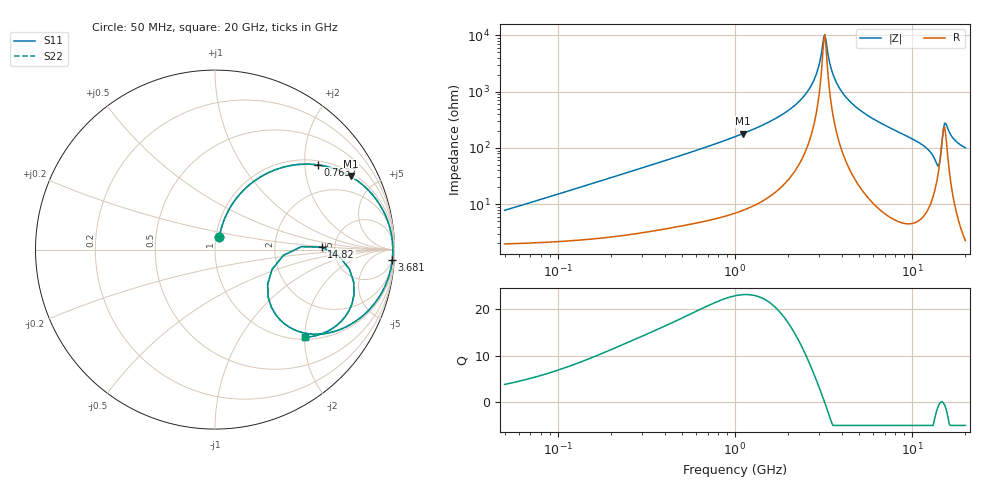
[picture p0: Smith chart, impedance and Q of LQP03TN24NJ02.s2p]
!Murata Part Number: LQP03TN24NJ02
!These Parameters are Measured in Series Mode Connection
!  o--[Z]--o
!Port1  Port2
!  o-------o
!Freq. Start=50[MHz] Stop=20[GHz], 401[Steps]
# Hz S RI R 50
!Freq.(Hz) S11(Real) S11(Imag) S21(Real) S21(Imag) S12(Real) S12(Imag) S22(Real) S22(Imag)
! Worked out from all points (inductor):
!   401 points, 50 MHz to 20 GHz, reference 50 ohm
!   read as one part in series: L = 23.9 nH near 51.52 MHz
!   highest Q = 23.2 at 1.111 GHz (marker M1), where L = 25.8 nH
!   self-resonance near 3.169 GHz
!   S11 on the Smith chart (normalised r, x): 50 MHz: 1.04, +0.15; 763.7 MHz: 1.11, +2.33; 3.681 GHz: 6, -32; 14.82 GHz: 3.94, +0.17; 20 GHz: 1.04, -2.01
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5e7  0.0246 0.072  0.9754 -0.072  0.9754 -0.072  0.0246 0.072
1.364002e8  0.0596 0.1864  0.9404 -0.1864  0.9404 -0.1864  0.0596 0.1864
3.721004e8  0.2461 0.4003  0.7539 -0.4003  0.7539 -0.4003  0.2461 0.4003
7.636728e8  0.572 0.472  0.428 -0.472  0.428 -0.472  0.572 0.472
1e9  0.7074 0.4337  0.2926 -0.4337  0.2926 -0.4337  0.7074 0.4337
1.110545e9  0.7557 0.4086  0.2443 -0.4086  0.2443 -0.4086  0.7557 0.4086
1.99176e9  0.9443 0.2021  0.0557 -0.2021  0.0557 -0.2021  0.9443 0.2021
2.728004e9  0.985 0.0696  0.015 -0.0696  0.015 -0.0696  0.985 0.0696
2.896447e9  0.9882 0.0439  0.0118 -0.0439  0.0118 -0.0439  0.9882 0.0439
3.121702e9  0.9904 0.0116  0.00965 -0.0116  0.00965 -0.0116  0.9904 0.0116
3.216634e9  0.9906 -0.00132  0.00941 0.00132  0.00941 0.00132  0.9906 -0.00132
3.680849e9  0.9873 -0.0598  0.0127 0.0598  0.0127 0.0598  0.9873 -0.0598
4.748272e9  0.9609 -0.1705  0.0391 0.1705  0.0391 0.1705  0.9609 -0.1705
7.442007e9  0.8355 -0.3581  0.1645 0.3581  0.1645 0.3581  0.8355 -0.3581
1.238412e10  0.4626 -0.4549  0.5374 0.4549  0.5374 0.4549  0.4626 -0.4549
1.314879e10  0.3645 -0.3935  0.6355 0.3935  0.6355 0.3935  0.3645 -0.3935
1.396067e10  0.2933 -0.193  0.7067 0.193  0.7067 0.193  0.2933 -0.193
1.482269e10  0.5954 0.0142  0.4046 -0.0142  0.4046 -0.0142  0.5954 0.0142
1.527346e10  0.7489 -0.1089  0.2511 0.1089  0.2511 0.1089  0.7489 -0.1089
1.573793e10  0.775 -0.2487  0.225 0.2487  0.225 0.2487  0.775 -0.2487
1.721783e10  0.6617 -0.4348  0.3383 0.4348  0.3383 0.4348  0.6617 -0.4348
2e10  0.5032 -0.489  0.4968 0.489  0.4968 0.489  0.5032 -0.489
